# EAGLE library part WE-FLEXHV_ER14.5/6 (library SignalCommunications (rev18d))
WE-FLEX HV Flexible Transformer for DC/DC Converter Characteristics Transformer with 6 identical windings 4 sizes with 5 different lengths of air gap each Isolation voltage up to 1.5 kVAC Low leakage inductance Operating temperature: –40 ºC to +125 ºC By using different circuits more than 375 transformer solutions and about 125 choke solutions possible. Consequently, quick prototyping possibilities EFD size parts provide Basic insulation for a working voltage of 250VRMS when they are connteced approbiate Applications Flyback converters Forward converters Push-pull converters Step-up/step-down converters SEPIC Details see: http://katalog.we-online.de/en/pbs/WE-FLEXHV/749196308?m Created by Yingchun Shan 2017 (C) Wurth Elektronik
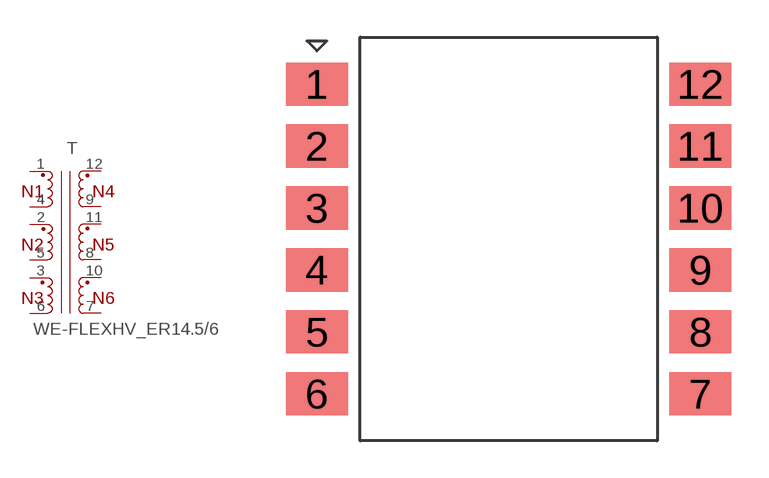
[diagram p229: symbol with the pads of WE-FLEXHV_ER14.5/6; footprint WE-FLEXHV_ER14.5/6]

Designator prefix T

## WE-FLEXHV_ER14.5/6_749196208 (WE-NUMBER: 749196208/165uH), WE-FLEXHV_ER14.5/6_749196218 (WE-NUMBER: 749196218/21,6uH), WE-FLEXHV_ER14.5/6_749196228 (WE-NUMBER: 749196228/11,6uH), WE-FLEXHV_ER14.5/6_749196238 (WE-NUMBER: 749196238/8,3uH), WE-FLEXHV_ER14.5/6_749196248 (WE-NUMBER: 749196248/6,6uH)  [WE-FLEXHV_ER14.5/6]
1  1  pas
2  2  pas
3  3  pas
4  4  pas
5  5  pas
6  6  pas
7  7  pas
8  8  pas
9  9  pas
10  10  pas
11  11  pas
12  12  pas

## Footprint WE-FLEXHV_ER14.5/6 (pad centres in mm)
smd 2.5 x 1.75: 1 -7.75,6.25; 2 -7.75,3.75; 3 -7.75,1.25; 4 -7.75,-1.25; 5 -7.75,-3.75; 6 -7.75,-6.25; 7 7.75,-6.25; 8 7.75,-3.75; 9 7.75,-1.25; 10 7.75,1.25; 11 7.75,3.75; 12 7.75,6.25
